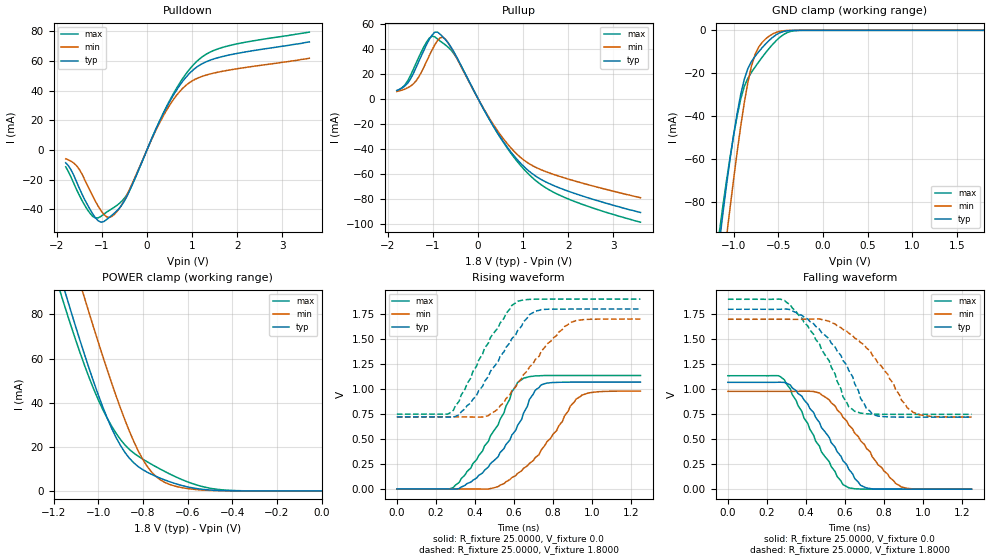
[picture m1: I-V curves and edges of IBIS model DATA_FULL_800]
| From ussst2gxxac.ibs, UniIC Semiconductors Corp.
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|If RDQS is enabled, then DM_RDQS is OUTPUT only (DATA_FULL and DATA_REDUCED)
|If RDQS is disabled, then DM_RDQS is INPUT
|with ODT(DATA_RCV/ODT_50/ODT_75/ODT150)
|   Model DATA_FULL_800
[Model]  DATA_FULL_800
Model_type I/O
Polarity   Non-Inverting
Enable   Active-High
Vinl =   0.70000000V
Vinh =   1.10000000V
Vmeas =   0.90000000V
Rref =   25.00000000
Vref =   0.90000000V
C_comp   2.5240pF   2.5060pF   2.5510pF
[Temperature Range]   25.0000   95.0000   0.0
[Voltage Range]   1.8000V   1.7000V   1.9000V
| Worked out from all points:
|   slope of the pulldown table from 0 to 0.27 V, typ, clamps not added: 14.5 ohm
|   slope of the pullup table from 0 to 0.27 V, typ, clamps not added: 15.2 ohm
|   GND clamp passes 1 mA (typ) near -0.47 V on its own axis
|   POWER clamp passes 1 mA (typ) near -0.55 V on its own axis
|   rising waveform, R_fixture 25.0000, V_fixture 0.0: 20-80 % time 208ps typ, 235ps min, 197ps max; typ from 0 V to 1.07 V
|   rising waveform, R_fixture 25.0000, V_fixture 1.8000: 20-80 % time 211ps typ, 232ps min, 191ps max; typ from 0.72 V to 1.8 V
|   falling waveform, R_fixture 25.0000, V_fixture 0.0: 20-80 % time 209ps typ, 230ps min, 187ps max; typ from 1.07 V to 0 V
|   falling waveform, R_fixture 25.0000, V_fixture 1.8000: 20-80 % time 202ps typ, 227ps min, 192ps max; typ from 1.8 V to 0.72 V
[Pulldown]
|Voltage   I(typ)   I(min)   I(max)
-1.8V     -8.6mA     -5.9mA     -11.3mA
-1.56V    -21.4mA    -10.5mA    -26.6mA
-1.26V    -40mA      -27.5mA    -42.6mA
-1.14V    -45.63mA   -34.6mA    -45.75mA
-960mV    -48.21mA   -43.16mA   -43.31mA
-720mV    -42.43mA   -43.22mA   -38.43mA
-420mV    -29.74mA   -28.8mA    -28.89mA
420mV     27.8mA     25.95mA    28.32mA
720mV     43.17mA    39.09mA    44.68mA
1.02V     53.74mA    46.78mA    56.97mA
1.68V     62.9mA     52.98mA    69.04mA
3.6V      72.7mA     61.7mA     79.3mA
[Pullup]
|Voltage   I(typ)   I(min)   I(max)
-1.8V     6.5mA      5.7mA      6.3mA
-1.62V    10.1mA     7.6mA      11mA
-1.38V    24.4mA     13.9mA     27.8mA
-1.08V    47.43mA    34.44mA    48.41mA
-900mV    53.26mA    46.36mA    47.78mA
-780mV    49.42mA    49.09mA    44.52mA
-660mV    44.42mA    44.58mA    41.07mA
-420mV    29.63mA    28.82mA    29.17mA
360mV     -23.16mA   -21.82mA   -23.39mA
1.08V     -56.49mA   -50.84mA   -58.95mA
1.86V     -72.23mA   -62.83mA   -78.14mA
3.6V      -91.1mA    -79.3mA    -98.9mA
[GND_clamp]
|Voltage   I(typ)   I(min)   I(max)
-1.8V     -341.4mA   -368.9mA   -332.4mA
-1.16V    -98.84mA   -124.9mA   -94.02mA
-1.12V    -85.23mA   -110.5mA   -81.66mA
-1.08V    -72.2mA    -96.41mA   -70.06mA
-1.04V    -59.93mA   -82.62mA   -59.18mA
-920mV    -29.77mA   -44.48mA   -31.9mA
-880mV    -22.69mA   -33.57mA   -26.06mA
-800mV    -14.49mA   -16.62mA   -19.53mA
-720mV    -10.02mA   -7.817mA   -14.76mA
-560mV    -3.159mA   -1.628mA   -6.393mA
-280mV    -8.14uA    -3.578uA   -70uA
1.8V      7.234nA    32.16nA    61.22nA
[POWER_clamp]
|Voltage   I(typ)   I(min)   I(max)
-1.8V     325.1mA    352.4mA    316.2mA
-1.16V    94.14mA    121mA      86.98mA
-1.14V    87.41mA    114.1mA    80.57mA
-1.06V    61.46mA    87.09mA    56.62mA
-980mV    38.21mA    61.22mA    37.03mA
-900mV    20.56mA    37.47mA    23.27mA
-820mV    10.96mA    18mA       15.69mA
-780mV    8.467mA    11.05mA    13.18mA
-740mV    6.55mA     6.435mA    10.88mA
-640mV    2.87mA     1.791mA    5.795mA
-480mV    290.4uA    171.3uA    911.2uA
0V        7.234nA    10.13nA    70.66nA
[Ramp]
| variable   typ   min   max
dV/dt_r  0.6414/0.2041n   0.5873/0.2469n   0.6810/0.1907n
dV/dt_f  0.6478/0.1974n   0.5871/0.2419n   0.6907/0.1840n
R_load = 25.0000
[Rising Waveform]
R_fixture= 25.0000
V_fixture= 0.0
V_fixture_min= 0.0
V_fixture_max= 0.0
|time   V(typ)   V(min)   V(max)
0s        0V         0V         0V
270ps     -505.2uV   -5.714uV   404.8uV
320ps     4.221mV    28.75uV    65.51mV
520ps     322.6mV    23.92mV    642.2mV
590ps     538.8mV    113.5mV    971.6mV
650ps     758.6mV    206.3mV    1.108V
740ps     1.041V     387.9mV    1.133V
890ps     1.069V     828.5mV    1.135V
950ps     1.069V     939.4mV    1.135V
1.25ns    1.069V     978.7mV    1.135V
[Rising Waveform]
R_fixture= 25.0000
V_fixture= 1.8000
V_fixture_min= 1.7000
V_fixture_max= 1.9000
|time   V(typ)   V(min)   V(max)
0s        720.4mV    721.5mV    748.8mV
260ps     719.1mV    721.5mV    748.6mV
290ps     720.1mV    721.5mV    786.8mV
380ps     861.2mV    720.2mV    1.11V
470ps     1.126V     733.6mV    1.46V
560ps     1.417V     903.3mV    1.755V
620ps     1.585V     1.061V     1.878V
710ps     1.779V     1.294V     1.899V
890ps     1.8V       1.665V     1.9V
1.25ns    1.8V       1.7V       1.9V
[Falling Waveform]
R_fixture= 25.0000
V_fixture= 0.0
V_fixture_min= 0.0
V_fixture_max= 0.0
|time   V(typ)   V(min)   V(max)
0s        1.069V     978.8mV    1.135V
260ps     1.07V      978.7mV    1.135V
290ps     1.068V     978.7mV    1.094V
380ps     929mV      979.5mV    775.7mV
470ps     665.9mV    961.9mV    429.4mV
560ps     376.1mV    794.7mV    127.8mV
620ps     199.2mV    642.5mV    13.31mV
710ps     12.03mV    409.1mV    368.8uV
890ps     5.526uV    21.53mV    0V
1.25ns    0V         0V         0V
[Falling Waveform]
R_fixture= 25.0000
V_fixture= 1.8000
V_fixture_min= 1.7000
V_fixture_max= 1.9000
|time   V(typ)   V(min)   V(max)
0s        1.8V       1.7V       1.9V
260ps     1.8V       1.7V       1.902V
320ps     1.797V     1.7V       1.845V
520ps     1.502V     1.679V     1.282V
590ps     1.288V     1.598V     925.3mV
650ps     1.057V     1.513V     779.2mV
680ps     910.4mV    1.468V     761.1mV
740ps     752.2mV    1.343V     750.4mV
950ps     720.5mV    769mV      748.8mV
1.25ns    720.4mV    721.5mV    748.8mV
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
